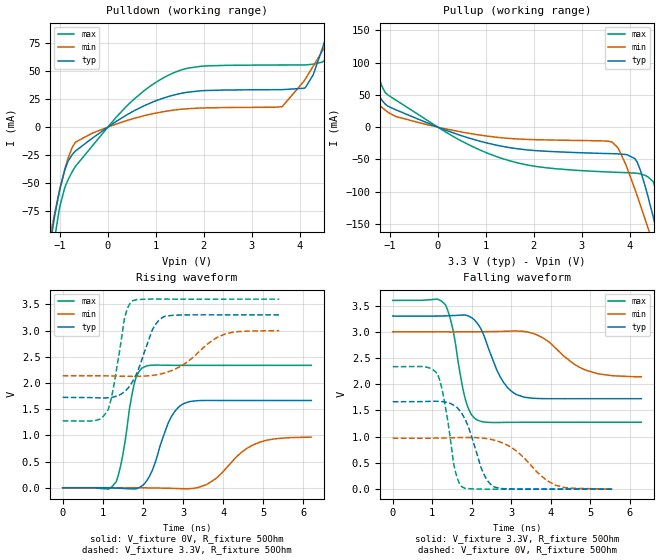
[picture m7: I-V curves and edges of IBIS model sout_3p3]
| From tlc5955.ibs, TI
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|   sout_3p3 Model
[Model]   sout_3p3
Model_type   Output
Polarity   Non-Inverting
Vmeas = 1.65
Vref = 0
Cref = 15pF
Rref = 100
|   typ   min   max
|   (nom PVT)   (fast PVT)   (slow PVT)
C_comp   1.371e-12   1.298e-12   1.531e-12
| Where nom  PVT is Nominal Process, 3.3V, 27C
|   Fast PVT is Strong Process,  3.6V, -40C
|   Slow PVT is Weak Process,   3V, 125C
[Voltage Range]   3.3   3   3.6
|Junction Temperature
[Temperature Range]   27   125   -40
[Pullup Reference]   3.3   3   3.6
[Pulldown Reference]   0   0   0
[Power Clamp Reference]   3.3   3   3.6
[GND Clamp Reference]   0   0   0
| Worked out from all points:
|   slope of the pulldown table from 0 to 0.495 V, typ, clamps not added: 37.1 ohm
|   slope of the pullup table from 0 to 0.495 V, typ, clamps not added: 37.2 ohm
|   falling waveform, V_fixture 3.3V, R_fixture 50Ohm: 20-80 % time 524ps typ, 839ps min, 334ps max; typ from 3.3 V to 1.73 V
|   rising waveform, V_fixture 0V, R_fixture 50Ohm: 20-80 % time 460ps typ, 798ps min, 293ps max; typ from 0 V to 1.67 V
|   rising waveform, V_fixture 3.3V, R_fixture 50Ohm: 20-80 % time 470ps typ, 848ps min, 301ps max; typ from 1.73 V to 3.3 V
|   falling waveform, V_fixture 0V, R_fixture 50Ohm: 20-80 % time 445ps typ, 815ps min, 289ps max; typ from 1.67 V to 0 V
[Pulldown]
|   Voltage   I(typ)   I(min)   I(max)
-3.3V     -791mA     -610.3mA   -1.126A
-1.37V    -154.2mA   -133.2mA   -215.9mA
-1.099V   -76.83mA   -74.75mA   -96.31mA
-880.8mV  -36.16mA   -34.92mA   -52.06mA
-675.6mV  -21.28mA   -13.38mA   -34.97mA
459mV     12.5mA     6.715mA    21.47mA
1.376V    28.59mA    15.18mA    48.45mA
3.633V    33.37mA    18.22mA    55.34mA
4.115V    35.05mA    42.78mA    55.42mA
4.478V    71.02mA    68.32mA    58.06mA
4.778V    111.5mA    89.94mA    112mA
6.6V      352.2mA    219.7mA    597.4mA
[Pullup]
|   Voltage   I(typ)   I(min)   I(max)
-3.3V     319mA      181.3mA    601.6mA
-2.029V   154.6mA    90.87mA    306.4mA
-1.331V   60.91mA    41.48mA    105.4mA
-873mV    26.77mA    16.39mA    41.79mA
1.326V    -29.51mA   -16.42mA   -48.25mA
3.634V    -41.12mA   -23.22mA   -69.74mA
4.112V    -49.03mA   -97.12mA   -71.19mA
4.382V    -108.2mA   -156.7mA   -77.38mA
4.577V    -165.4mA   -201.7mA   -105mA
4.678V    -196.5mA   -225.5mA   -145.2mA
4.825V    -243.1mA   -260.8mA   -213.2mA
6.6V      -834.9mA   -710.7mA   -1.07A
[Ramp]
R_load = 50
|   typ   min   max
dV/dt_r   0.999432/4.57494e-10   0.58229/7.968e-10   1.40136/2.91764e-10
dV/dt_f   0.945123/5.23253e-10   0.517403/8.45869e-10   1.39473/3.33086e-10
[Falling Waveform]
V_fixture = 3.3V
V_fixture_min = 3V
V_fixture_max = 3.6V
R_fixture = 50Ohm
|   Time   V(typ)   V(min)   V(max)
0s        3.3V       3V         3.6V
1.334ns   3.304V     3V         3.518V
1.534ns   3.311V     3V         3.007V
1.844ns   3.319V     3V         1.699V
2.133ns   3.17V      3.001V     1.319V
2.714ns   2.151V     3.008V     1.271V
3.146ns   1.799V     3.016V     1.275V
3.788ns   1.726V     2.89V      1.276V
4.879ns   1.725V     2.271V     1.275V
6.29ns    1.725V     2.144V     1.275V
[Rising Waveform]
V_fixture = 0V
V_fixture_min = 0V
V_fixture_max = 0V
R_fixture = 50Ohm
|   Time   V(typ)   V(min)   V(max)
0s        1.217nV    7.603nV    889.5pV
1.334ns   -6.573mV   552.6uV    114.7mV
1.495ns   -12.47mV   563.2uV    612.8mV
1.786ns   -21.28mV   -70.09uV   1.996V
1.976ns   36.17mV    -1.278mV   2.284V
2.711ns   1.359V     -11.24mV   2.337V
2.989ns   1.595V     -18.32mV   2.336V
3.62ns    1.666V     74.66mV    2.336V
4.916ns   1.666V     870.7mV    2.336V
6.198ns   1.666V     966.5mV    2.336V
[Rising Waveform]
V_fixture = 3.3V
V_fixture_min = 3V
V_fixture_max = 3.6V
R_fixture = 50Ohm
|   Time   V(typ)   V(min)   V(max)
0s        1.725V     2.138V     1.276V
834ps     1.717V     2.137V     1.287V
1.134ns   1.718V     2.135V     1.492V
1.278ns   1.734V     2.133V     1.966V
1.535ns   1.832V     2.129V     3.212V
1.75ns    2.038V     2.126V     3.572V
2.226ns   2.996V     2.143V     3.601V
2.495ns   3.254V     2.182V     3.601V
4.059ns   3.3V       2.94V      3.6V
5.399ns   3.3V       2.999V     3.6V
[Falling Waveform]
V_fixture = 0V
V_fixture_min = 0V
V_fixture_max = 0V
R_fixture = 50Ohm
|   Time   V(typ)   V(min)   V(max)
0s        1.666V     970.6mV    2.336V
1.134ns   1.675V     973.9mV    2.199V
1.314ns   1.662V     976.3mV    1.655V
1.534ns   1.604V     980mV      511.9mV
1.746ns   1.444V     983.5mV    47.13mV
2.277ns   333.5mV    973mV      -101.5uV
2.568ns   42.6mV     934.4mV    -549.9uV
3.053ns   4.058mV    769.3mV    2.192uV
4.121ns   21.5uV     74.28mV    29.04uV
5.554ns   52.53uV    2.056mV    13.56uV
